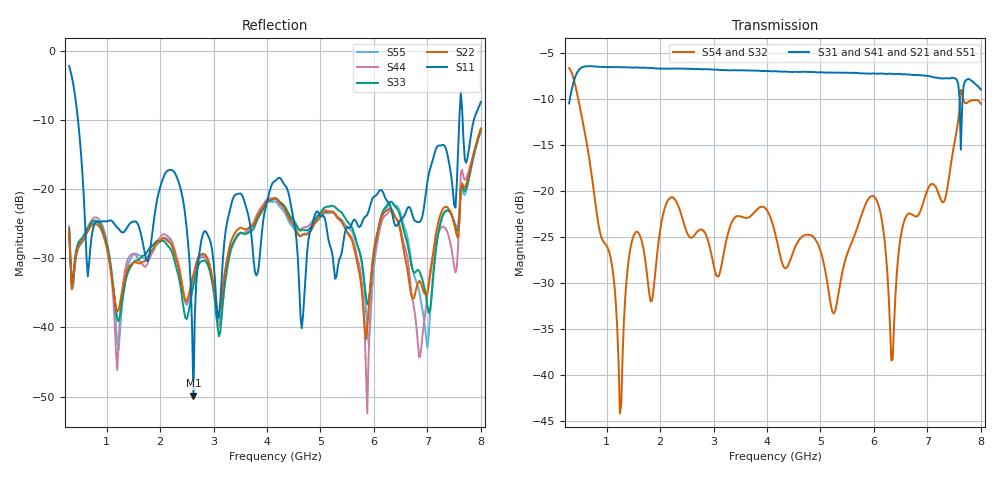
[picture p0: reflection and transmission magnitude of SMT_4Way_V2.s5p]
! Created Tue Jan 09 16:32:45 2018
# hz S ma R 50
! 5 Port Network Data from SP1.SP block
! freq  magS11  angS11  magS12  angS12  magS13  angS13  magS14  angS14
!  magS15  angS15
!  magS21  angS21  magS22  angS22  magS23  angS23
!  magS24  angS24  magS25  angS25
!  magS31  angS31  magS32  angS32
!  magS33  angS33  magS34  angS34  magS35  angS35
!  magS41  angS41
!  magS42  angS42  magS43  angS43  magS44  angS44  magS45  angS45
!  magS51  angS51  magS52  angS52  magS53  angS53  magS54  angS54
!  magS55  angS55
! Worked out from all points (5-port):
!   309 points, 300 MHz to 8 GHz, reference 50 ohm
!   strongest paths, dB at 300 MHz, 2.225 GHz, 4.15 GHz, 6.075 GHz, 8 GHz:
!     S31: -10.4, -6.7, -7.0, -7.2, -8.9
!     S41: -10.5, -6.7, -7.0, -7.3, -9.0
!     S21: -10.4, -6.7, -7.0, -7.3, -8.9
!     S51: -10.5, -6.7, -7.0, -7.3, -9.0
!     S54: -6.6, -20.6, -24.5, -21.4, -10.5
!     S32: -6.6, -20.6, -24.5, -21.4, -10.5
!   lowest |S11| = -49.9 dB at 2.625 GHz (marker M1), VSWR 1.01, Z = 50 - j0.319 ohm
!   |S11| at or under -10 dB: 466.1 MHz to 7.597 GHz (7.131 GHz wide, 177 % of centre); 7.659 GHz to 7.868 GHz (208.8 MHz wide, 2.69 % of centre)
